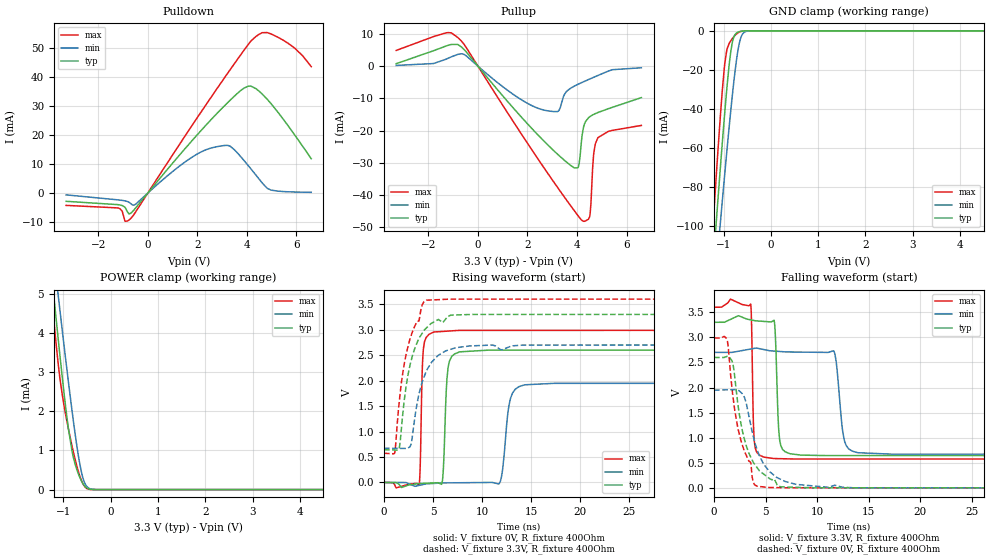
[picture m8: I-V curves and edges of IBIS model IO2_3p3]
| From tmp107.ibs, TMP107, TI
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|   Model
[Model]   IO2_3p3
Model_type   I/O
Polarity   Non-Inverting
Enable   Active-Low
Vinl = 0.99
Vinh = 2.31
Vmeas = 1.65
Vref = 0
Cref = 1pF
Rref = 100000
|   typ   min   max
C_comp   1.060pF   1.035pF   1.082pF
[Voltage Range]   3.3   2.7   3.6
[Temperature Range]   25   125   -55
[Pullup Reference]   3.3   2.7   3.6
[Pulldown Reference]   0   0   -0
[Power Clamp Reference]   3.3   2.7   3.6
[GND Clamp Reference]   0   0   0
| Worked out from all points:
|   slope of the pulldown table from 0 to 0.495 V, typ, clamps not added: 96.5 ohm
|   slope of the pullup table from 0 to 0.495 V, typ, clamps not added: 107 ohm
|   GND clamp passes 1 mA (typ) near -0.72 V on its own axis
|   POWER clamp passes 1 mA (typ) near -0.82 V on its own axis
|   falling waveform, V_fixture 3.3V, R_fixture 400Ohm: 20-80 % time 271ps typ, 561ps min, 172ps max; typ from 3.3 V to 0.643 V
|   rising waveform, V_fixture 0V, R_fixture 400Ohm: 20-80 % time 330ps typ, 624ps min, 212ps max; typ from 0 V to 2.6 V
|   rising waveform, V_fixture 3.3V, R_fixture 400Ohm: 20-80 % time 1.6ns typ, 1.63ns min, 1.6ns max; typ from 0.643 V to 3.3 V
|   falling waveform, V_fixture 0V, R_fixture 400Ohm: 20-80 % time 1.7ns typ, 1.87ns min, 1.69ns max; typ from 2.6 V to 0 V
[Pulldown]
|   Voltage   I(typ)   I(min)   I(max)
-3.3V     -2.841mA   -618.4uA   -4.245mA
-1.211V   -3.984mA   -2.334mA   -5.111mA
-914.1mV  -4.968mA   -2.702mA   -9.725mA
-755.7mV  -7.198mA   -3.174mA   -9.255mA
-518.1mV  -5.402mA   -3.975mA   -6.838mA
1.393V    14.19mA    10.01mA    18.21mA
2.511V    24.89mA    15.39mA    32.45mA
3.313V    31.89mA    16.18mA    42.35mA
4.046V    36.78mA    9.568mA    51.08mA
4.828V    32.26mA    1.619mA    55.26mA
5.917V    20.2mA     368.3uA    50.02mA
6.6V      11.84mA    257.3uA    43.55mA
[GND Clamp]
|   Voltage   I(typ)   I(min)   I(max)
-3.3V     -846.7mA   -754.5mA   -933.2mA
-1.32V    -153.2mA   -169.4mA   -137.1mA
-1.201V   -113.5mA   -135.7mA   -91.8mA
-1.181V   -107mA     -130.1mA   -84.42mA
-1.122V   -87.61mA   -113.5mA   -62.75mA
-1.073V   -71.78mA   -99.83mA   -45.51mA
-973.5mV  -41.63mA   -73.07mA   -16.75mA
-844.8mV  -10.28mA   -40.31mA   -4.995mA
-686.4mV  -594.7uA   -8.806mA   -920.2uA
-597.3mV  -116.8uA   -1.62mA    -164.4uA
-448.8mV  -3.867uA   -44uA      -2.799uA
6.6V      0A         0A         0A
[Pullup]
|   Voltage   I(typ)   I(min)   I(max)
-3.3V     769.3uA    225uA      4.88mA
-815.1mV  6.75mA     3.651mA    8.909mA
2.65V     -23.14mA   -13.61mA   -31.36mA
3.244V    -27.55mA   -13.97mA   -37.96mA
3.551V    -29.61mA   -8.115mA   -41.28mA
3.897V    -31.62mA   -6.183mA   -44.94mA
4.085V    -30.39mA   -5.474mA   -46.88mA
4.264V    -18.95mA   -4.846mA   -48.18mA
4.521V    -15.68mA   -3.972mA   -46.38mA
4.67V     -15mA      -3.476mA   -27.65mA
4.838V    -14.42mA   -2.918mA   -22.3mA
6.6V      -9.766mA   -496uA     -18.4mA
[POWER Clamp]
|   Voltage   I(typ)   I(min)   I(max)
-3.3V     31.68mA    29.28mA    35.71mA
-1.28V    5.915mA    6.809mA    5.409mA
-1.162V   4.483mA    5.539mA    3.842mA
-1.102V   3.786mA    4.911mA    3.156mA
-1.003V   2.669mA    3.879mA    2.279mA
-943.8mV  2.048mA    3.273mA    1.876mA
-815.1mV  981.8uA    2.014mA    1.111mA
-745.8mV  634.6uA    1.388mA    753.2uA
-646.8mV  301.1uA    628.9uA    333.3uA
-567.6mV  124.3uA    232.8uA    112.4uA
-488.4mV  32.9uA     61.81uA    19.85uA
6.6V      0A         0A         0A
[Ramp]
R_load = 400
|   typ   min   max
dV/dt_r   1.55918/3.23323e-10   1.16844/6.12056e-10   1.79224/2.10051e-10
dV/dt_f   1.59447/2.69552e-10   1.21733/5.55777e-10   1.81552/1.70784e-10
[Falling Waveform]
V_fixture = 3.3V
V_fixture_min = 2.7V
V_fixture_max = 3.6V
R_fixture = 400Ohm
C_fixture = 0F
|   Time   V(typ)   V(min)   V(max)
0s        3.3V       2.7V       3.6V
3.548ns   3.349V     2.767V     3.663V
3.902ns   3.334V     2.78V      936.3mV
4.811ns   3.318V     2.757V     614.3mV
5.827ns   3.335V     2.726V     584.3mV
6.349ns   977.6mV    2.719V     582mV
7.35ns    681.4mV    2.708V     577.4mV
11.62ns   643.5mV    2.724V     574.8mV
13.9ns    643.4mV    702.5mV    574.7mV
50ns      642.5mV    671.1mV    574.1mV
[Rising Waveform]
V_fixture = 0V
V_fixture_min = 0V
V_fixture_max = 0V
R_fixture = 400Ohm
C_fixture = 0F
|   Time   V(typ)   V(min)   V(max)
0s        131nV      194.9nV    101.9nV
3.578ns   -21.22mV   -58.46mV   -51.78mV
4.024ns   -17.41mV   -39.31mV   2.616V
5.102ns   -8.395mV   -19.03mV   2.955V
5.969ns   38.96mV    -9.079mV   2.965V
6.569ns   2.284V     -7.825mV   2.973V
7.698ns   2.563V     -5.683mV   2.986V
11.76ns   2.598V     -22.51mV   2.987V
14.34ns   2.598V     1.917V     2.987V
50ns      2.599V     1.947V     2.987V
[Rising Waveform]
V_fixture = 3.3V
V_fixture_min = 2.7V
V_fixture_max = 3.6V
R_fixture = 400Ohm
C_fixture = 0F
|   Time   V(typ)   V(min)   V(max)
0s        642.5mV    671.1mV    574.1mV
1.101ns   637.1mV    669.4mV    581mV
1.558ns   666.7mV    668.7mV    1.575V
2.078ns   1.626V     667.9mV    2.333V
2.654ns   2.299V     698.5mV    2.814V
3.531ns   2.811V     1.7V       3.169V
4.318ns   3.031V     2.183V     3.579V
6.283ns   3.205V     2.583V     3.596V
8.741ns   3.298V     2.681V     3.6V
50ns      3.3V       2.7V       3.6V
[Falling Waveform]
|Gnd
V_fixture = 0V
V_fixture_min = 0V
V_fixture_max = 0V
R_fixture = 400Ohm
C_fixture = 0F
|   Time   V(typ)   V(min)   V(max)
0s        2.599V     1.947V     2.987V
1.272ns   2.621V     1.954V     2.94V
1.826ns   2.473V     1.957V     1.824V
2.296ns   1.687V     1.946V     1.206V
3.105ns   850.3mV    1.698V     657.8mV
3.8ns     510.7mV    1.032V     108.7mV
4.175ns   402.4mV    764.5mV    33.19mV
6.054ns   86.85mV    210.2mV    5.068mV
11.06ns   461.1uV    11.96mV    559uV
50ns      316.6nV    393nV      232.2nV
